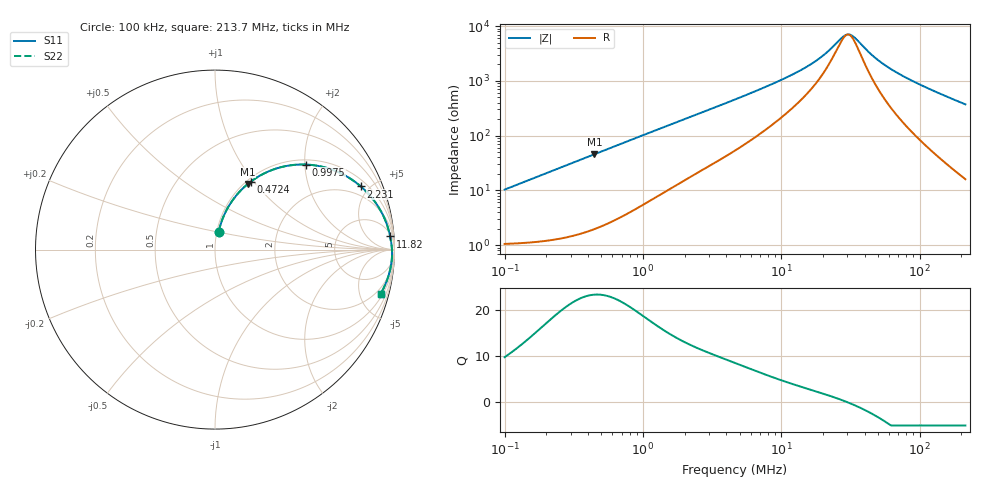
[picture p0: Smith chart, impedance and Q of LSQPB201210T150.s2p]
! LSQPB201210T150  S-PARAMETER MODEL  ( General Type )
! Model Generated by TAIYO YUDEN Corporation (http://www.ty-top.com)
! Version 2.0
! TAIYO YUDEN Control No. 100810NF18SB-HKC
! Copyright(c) 2007 TAIYO YUDEN CO.,LTD. All Rights Reserved.
! Product Description (link to TY-COMPAS)
! https://ds.yuden.co.jp/TYCOMPAS/or/detail?pn=LSQPB201210T150M&u=M
! Products Name : Inductors
! Characteristics :
!  Inductance : 15 uH , SRF(min) : 15 MHz , DC Resistance(max) : 1.3 Ohm
!  Rated Current : Saturation :220 mA , Temp Rise : 300 mA (40 degC)
!  Case Size : 2.0 x 1.25 / 0.079 x 0.049 [mm/inch] , Thickness : 1.0 / 0.04 [mm/inch]
!  (Conditions: Temperature = 25 degC , DC Bias Current/Voltage = 0A / 0V)
! External Node Assignments :
!  1  o---GGG---o  2
! GND o---------o GND
! Frequency Range : 0.1MHz  -  213.673535MHz  [ 402 STEP ]
# MHz S RI R 50
! Freq[MHz].  S11 Real  S11 Imag  S21 Real  S21 Imag  S12 Real  S12 Imag  S22 Real  S22 Imag
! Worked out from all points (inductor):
!   401 points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, 100 kHz to 213.7 MHz, reference 50 ohm
!   read as one part in series: L = 16.3 uH near 103.9 kHz
!   highest Q = 23.3 at 446 kHz (marker M1), where L = 16.3 uH
!   self-resonance near 30.15 MHz
!   S11 on the Smith chart (normalised r, x): 100 kHz: 1.02, +0.20; 472.4 kHz: 1.04, +0.96; 997.5 kHz: 1.11, +2.02; 2.231 MHz: 1.36, +4.43; 11.82 MHz: 7, +25; 213.7 MHz: 1.32, -7.41
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0.1  0.0204 0.0993  0.9796 -0.0993  0.9796 -0.0993  0.0204 0.0993
0.211179  0.0551 0.2018  0.9449 -0.2018  0.9449 -0.2018  0.0551 0.2018
0.361188  0.1308 0.3158  0.8692 -0.3158  0.8692 -0.3158  0.1308 0.3158
0.445966  0.1825 0.3653  0.8175 -0.3653  0.8175 -0.3653  0.1825 0.3653
0.472362  0.1992 0.3785  0.8008 -0.3785  0.8008 -0.3785  0.1992 0.3785
0.706458  0.3481 0.4538  0.6519 -0.4538  0.6519 -0.4538  0.3481 0.4538
0.997528  0.5057 0.4739  0.4943 -0.4739  0.4943 -0.4739  0.5057 0.4739
1.304567  0.6267 0.4539  0.3733 -0.4539  0.3733 -0.4539  0.6267 0.4539
2.231254  0.8124 0.3519  0.1876 -0.3519  0.1876 -0.3519  0.8124 0.3519
3.150561  0.8849 0.2748  0.1151 -0.2748  0.1151 -0.2748  0.8849 0.2748
4.71194  0.9345 0.195  0.0655 -0.195  0.0655 -0.195  0.9345 0.195
7.90602  0.9652 0.1169  0.0348 -0.1169  0.0348 -0.1169  0.9652 0.1169
11.82415  0.976 0.073  0.024 -0.073  0.024 -0.073  0.976 0.073
16.69585  0.9812 0.0434  0.0188 -0.0434  0.0188 -0.0434  0.9812 0.0434
21.01363  0.9835 0.026  0.0165 -0.026  0.0165 -0.026  0.9835 0.026
28.01346  0.9856 0.00529  0.0144 -0.00529  0.0144 -0.00529  0.9856 0.00529
30.83107  0.986 -0.00162  0.014 0.00162  0.014 0.00162  0.986 -0.00162
33.28788  0.9863 -0.00722  0.0137 0.00722  0.0137 0.00722  0.9863 -0.00722
46.11058  0.9864 -0.0323  0.0136 0.0323  0.0136 0.0323  0.9864 -0.0323
60.30341  0.985 -0.0558  0.015 0.0558  0.015 0.0558  0.985 -0.0558
103.1394  0.9749 -0.1164  0.0251 0.1164  0.0251 0.1164  0.9749 -0.1164
213.6735  0.9231 -0.2458  0.0769 0.2458  0.0769 0.2458  0.9231 -0.2458
